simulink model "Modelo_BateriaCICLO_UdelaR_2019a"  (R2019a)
settings: Solver=VariableStepAuto  StartTime=0.0  StopTime=inf  RelTol=1e-3
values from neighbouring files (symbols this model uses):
  a = x(1)    [Cycling_LiFePO4.m]    (also in Parametros_A123.m = 2.09162011618e-08; Parametros_A123_pack.m = 2.09162011618e-08)
  A = @(x) x(1)    [Cycling_LiFePO4.m]    (also in LMFsolve.m = J'*J; Parametros_A123.m = 0.3446; Parametros_A123_pack.m = 0.3446)
  Alpha = 1093.6    [Parametros_A123.m]    (also in Parametros_A123_pack.m)
  b = x(2)    [Cycling_LiFePO4.m]    (also in Parametros_A123.m = -1.21794950859e-05; Parametros_A123_pack.m = -1.21794950859e-05)
  B = @(x) x(2)    [Cycling_LiFePO4.m]    (also in Parametros_A123.m = 13.0435; Parametros_A123_pack.m = 13.0435)
  Beta = 8390.6    [Parametros_A123.m]    (also in Parametros_A123_pack.m)
  c = x(3)    [Cycling_LiFePO4.m]    (also in Parametros_A123.m = 0.00180276688394; Parametros_A123_pack.m = 0.00180276688394)
  Cpol = 0    [Parametros_A123.m]    (also in Parametros_A123_pack.m)
  d = x(4)    [Cycling_LiFePO4.m]    (also in LMFsolve.m = (A+l*D)\v; Parametros_A123.m = -1.70817769928e-06; Parametros_A123_pack.m = -1.70817769928e-06)
  dE_dT = 0.000010001    (= 1.0001e-05)    [Parametros_A123.m]    (also in Parametros_A123_pack.m)
  dQ_dT = 0.0037    [Parametros_A123.m]    (also in Parametros_A123_pack.m)
  Eo = 3.3678    [Parametros_A123.m]    (also in Parametros_A123_pack.m)
  f = x(1)*Q0    [Calendar_LiFePO4.m]    (also in Cycling_LiFePO4.m = f*(exp(g)-1)/(g*exp(0.5)); LMFsolve.m = '; Parametros_A123.m = 5980801.16971; Parametros_A123_pack.m = 5980801.16971)
  g = x(2)    [Calendar_LiFePO4.m]    (also in Cycling_LiFePO4.m = 0.689770643187; Parametros_A123.m = 0.689770643187; Parametros_A123_pack.m = 0.689770643187)
  h = x(3)    [Calendar_LiFePO4.m]    (also in Cycling_LiFePO4.m = -6464.71191685; Parametros_A123.m = -6464.71191685; Parametros_A123_pack.m = -6464.71191685)
  K = 0.0029    [Parametros_A123.m]    (also in Parametros_A123_pack.m)
  Kc = 0.1    [Parametros_A123.m]    (also in Parametros_A123_pack.m)
  Np = 1    [Parametros_A123.m]    (also in Parametros_A123_pack.m = 10)
  Ns = 1    [Parametros_A123.m]    (also in Parametros_A123_pack.m = 200)
  Q = zeros(9,12)    [Calendar_LiFePO4.m]    (also in Cycling_LiFePO4.m = transpose(Q); Parametros_A123.m = 2.3; Parametros_A123_pack.m = 2.3)
  Rohm = 0.01    [Parametros_A123.m]    (also in Parametros_A123_pack.m)
  Rout = 0.6    [Parametros_A123.m]    (also in Parametros_A123_pack.m)
  SOC0 = 100    [Parametros_A123.m]    (also in Parametros_A123_pack.m)
  Ta = 45    [Parametros_A123.m]    (also in Parametros_A123_pack.m = 25)
  Tcrit = 65    [Parametros_A123.m]    (also in Parametros_A123_pack.m)
  Tf = 10    [Parametros_A123.m]    (also in Parametros_A123_pack.m)
  To = 298.15    [Parametros_A123.m]    (also in Parametros_A123_pack.m)
  Tth = 1000    [Parametros_A123.m]    (also in Parametros_A123_pack.m)
  w = 1.5    [Parametros_A123.m]    (also in Parametros_A123_pack.m)
undefined symbols (not defined in the file or in its folder): blocks, Continuous, kV, MW, nthroot, powergui, ZData
libraries: powerlib x8, simulink x3, simulink_extras x1

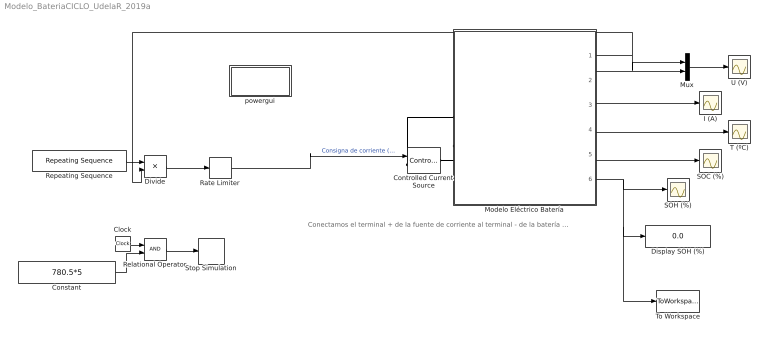
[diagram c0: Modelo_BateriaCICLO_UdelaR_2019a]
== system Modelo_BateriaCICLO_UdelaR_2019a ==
  note: Conectamos el terminal + de la fuente de corriente al terminal - de la batería y viceversa porque consideramos i > 0 durante la descarga.
  Clock : Clock
  Constant : Constant  Value=780.5*5
  Controlled Current Source : powerlib/Electrical Sources/Controlled Current Source  Initialize=on  Source_Type=AC  Amplitude=0  Phase=0  Frequency=0  Measurements=None
  Display SOH (%) : Display
  Divide : Product  Inputs=*/
  I (A) : Scope
  Modelo Eléctrico Batería : Subsystem  VariantControl=Continuous
  Mux : Mux  Inputs=2
  Rate Limiter : RateLimiter  RisingSlewLimit=inf  FallingSlewLimit=-inf  SampleTimeMode=inherited
  Relational Operator : RelationalOperator  OutDataTypeStr=boolean  RndMeth=Simplest
  Repeating Sequence : simulink/Sources/Repeating Sequence  rep_seq_t=t  rep_seq_y=P
  SOC (%) : Scope
  SOH (%) : Scope
  Stop Simulation : Stop
  T (ºC) : Scope
  To Workspace : ToWorkspace  VariableName=SOH  SampleTime=7000
  U (V) : Scope
  powergui : Subsystem  Priority=1  AncestorBlock=powerlib/powergui  DialogController=POWERSYS.PowerSysDialog  InitFcn=powergui( 'InitFcn_Callback' , gcb , 0 , [ ] );  mask(PSB option menu block){SimulationMode=Continuous, SampleTime=50e-6, frequency=60, Iterations=50, frequencyindice=0, Pbase=100e6, ErrMax=1e-4, UnitsV=kV, UnitsW=MW, buscounter=0, FunctionMessages=off, echomessages=off, EnableUseOfTLC=off, CurrentSourceSwitches=off, DisableSnubberDevices=off, DisableRonSwitches=off, DisableVfSwitches=off, DisplayEquations=off, AutomaticDiscreteSolvers=off, SolverType=Tustin/Backward Euler (TBE), Interpol=off, ExternalGateDelay=off, methode=off, Ts=100, x0status=blocks, SPID=on, SwTol=0, HookPort=off, NonlinearTolerance=1e-4, nMaxIteration=100, ContinueOnMaxIteration=off, RestoreLinks=warning, ResistiveCurrentMeasurement=off, Frange=[0:2:500], Ylog=off, Xlog=on, ShowGrid=off, save=off, variable=ZData, structure=0, ZoomFFT=off, StartTime=0.0, cycles=1, DisplayStyle=1, fundamental=60, FreqAxis=off, MaxFrequency=1000, frequencyindicesteady=1, RmsSteady=1, display=off}
      mask prompts: SimulationMode "Simulation type:"; SampleTime "Sample time (s):"; frequency "Frequency (Hz):"; Iterations "Max iterations"; frequencyindice "Frequency (Hz)"; Pbase "Base power (VA)"; ErrMax "PQ tolerance (pu)"; UnitsV "Voltage units"; UnitsW "Power units"; buscounter "Load flow bus counter"; FunctionMessages "Disable Specialized Power Systems warnings"; echomessages "Display Specialized Power Systems compilation messages"; EnableUseOfTLC "Use TLC file when in Accelerator Simulation Mode and for code generation"; CurrentSourceSwitches "Disable ideal switching"; DisableSnubberDevices "Disable snubbers in switching devices"; DisableRonSwitches "Disable Ron resistances in switching devices"; DisableVfSwitches "Disable forward voltages in switching devices"; DisplayEquations "Display circuit differential equations"; AutomaticDiscreteSolvers "Automatically handle Discrete solver and Advanced tab solver settings of blocks"; SolverType "Discrete solver"; Interpol "Interpolate switching events"; ExternalGateDelay "Use time-stamped gate signals"; methode "Store switching topologies"; Ts "Buffer size (MBytes):"; x0status "Start simulation with initial electrical states from:"; SPID "Use ideal switching devices"; SwTol "Switch tolerance"; HookPort "Allow multiple powergui blocks"; NonlinearTolerance "Solver tolerance"; nMaxIteration "Maximum number of iterations"; ContinueOnMaxIteration "Continue Simulation if maximum number of iterations is reached"; RestoreLinks "Restore disabled links of Simscape Power Systems ST blocks:"; ResistiveCurrentMeasurement "Use non ideal current measurement blocks (1e-4Ohm internal resistance)"; Frange "Frequency Range"; Ylog "Log impedance"; Xlog "log Frequency"; ShowGrid "grid"; save "Save Data To Workspace"; variable "Variable Name"; structure "Structure Name (PSBFFTSCOPE)"; ZoomFFT "ZoomFFT (PSBFFTSCOPE)"; StartTime "Start Time (PSBFFTSCOPE)"; cycles "Cycles (PSBFFTSCOPE)"; DisplayStyle "Display style (PSBFFTSCOPE)"; fundamental "Fundamental (PSBFFTSCOPE)"; FreqAxis "Frequency Axis (PSBFFTSCOPE)"; MaxFrequency "Max Frequency (PSBFFTSCOPE)"; frequencyindicesteady "Frequency indice (STEADYSTATE)"; RmsSteady "RMS display (STEADYSTATE)"; display "Display Results"
      mask help: Set simulation type, simulation parameters, and preferences.
      mask init:
      | dispMessage = powergui('MaskInitialization',gcb,SimulationMode,SampleTime);
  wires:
  Rate Limiter/1 -> Controlled Current Source/1  "Consigna de corriente (A)"
  Modelo Eléctrico Batería/5(SOC) -> SOC (%)/1
  Modelo Eléctrico Batería/6(SOH) -> SOH (%)/1, To Workspace/1, Display SOH (%)/1
  Modelo Eléctrico Batería/2(E) -> Mux/2
  Modelo Eléctrico Batería/3(I medida) -> I (A)/1
  Modelo Eléctrico Batería/4(T) -> T (ºC)/1
  Modelo Eléctrico Batería/1(U) -> Divide/2, Mux/1
  Mux/1 -> U (V)/1
  Repeating Sequence/1 -> Divide/1
  Divide/1 -> Rate Limiter/1
  Clock/1 -> Relational Operator/1
  Constant/1 -> Relational Operator/2
  Relational Operator/1 -> Stop Simulation/1
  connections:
  Modelo Eléctrico Batería/LConn2 -- Controlled Current Source/RConn1
  Modelo Eléctrico Batería/LConn1 -- Controlled Current Source/LConn1

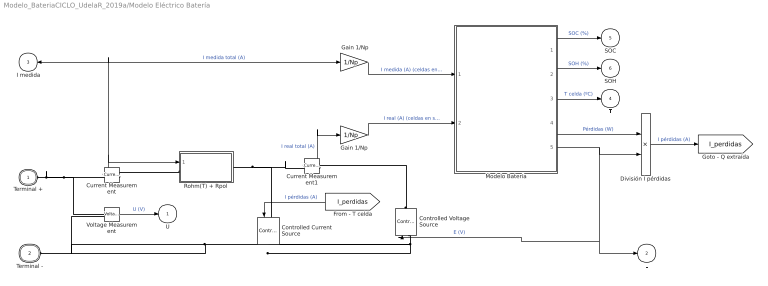
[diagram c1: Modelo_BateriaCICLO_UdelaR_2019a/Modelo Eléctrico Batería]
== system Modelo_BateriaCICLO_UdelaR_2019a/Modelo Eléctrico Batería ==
  "  Gain 1/Np " : Gain  Gain=1/Np
  " Gain 1/Np " : Gain  Gain=1/Np
  Controlled Current Source : powerlib/Electrical Sources/Controlled Current Source  Initialize=on  Source_Type=AC  Amplitude=0  Phase=0  Frequency=0  Measurements=None
  Controlled Voltage Source : powerlib/Electrical Sources/Controlled Voltage Source  Initialize=on  Source_Type=AC  Amplitude=0  Phase=0  Frequency=0  Measurements=None
  Current Measurement : powerlib/Measurements/Current Measurement  PhasorSimulation=off  OutputType=Complex  PSBequivalent=0
  Current Measurement1 : powerlib/Measurements/Current Measurement  PhasorSimulation=off  OutputType=Complex  PSBequivalent=0
  División I pérdidas : Product  Inputs=*/
  Modelo Batería : Subsystem  VariantControl=Continuous
  Rohm(T) + Rpol : Subsystem  VariantControl=Continuous
  Voltage Measurement : powerlib/Measurements/Voltage Measurement  PhasorSimulation=off  OutputType=Complex  PSBequivalent=0
  Terminal + : PMIOPort  Side=Left
  Terminal - : PMIOPort  Port=2  Side=Left
  U : Outport  VectorParamsAs1DForOutWhenUnconnected=off
  E : Outport  Port=2  VectorParamsAs1DForOutWhenUnconnected=off
  I medida : Outport  Port=3  VectorParamsAs1DForOutWhenUnconnected=off
  T : Outport  Port=4  VectorParamsAs1DForOutWhenUnconnected=off
  SOC : Outport  Port=5  VectorParamsAs1DForOutWhenUnconnected=off
  SOH : Outport  Port=6  VectorParamsAs1DForOutWhenUnconnected=off
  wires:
  Voltage Measurement/1 -> U/1  "U (V)"
  Current Measurement/1 -> "  Gain 1/Np "/1, I medida/1, Rohm(T) + Rpol/1(I medida)  "I medida total (A)"
  Current Measurement1/1 -> " Gain 1/Np "/1  "I real total (A)"
  [I_perdidas] -> Controlled Current Source/1  "I pérdidas (A)"
  Modelo Batería/1(SOC) -> SOC/1  "SOC (%)"
  Modelo Batería/2(SOH) -> SOH/1  "SOH (%)"
  Modelo Batería/3(T) -> T/1  "T celda (ºC)"
  Modelo Batería/5(E) -> División I pérdidas/2, Controlled Voltage Source/1, E/1  "E (V)"
  Modelo Batería/4(P Temp) -> División I pérdidas/1  "Pérdidas (W)"
  División I pérdidas/1 -> [I_perdidas]  "I pérdidas (A)"
  " Gain 1/Np "/1 -> Modelo Batería/2(I real)  "I real (A) (celdas en serie)"
  "  Gain 1/Np "/1 -> Modelo Batería/1(I medida)  "I medida (A) (celdas en serie)"
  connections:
  Terminal +/RConn1 -- Voltage Measurement/LConn1 -- Current Measurement/RConn1
  Controlled Voltage Source/LConn1 -- Controlled Current Source/RConn1 -- Voltage Measurement/LConn2 -- Terminal -/RConn1
  Current Measurement/LConn1 -- Rohm(T) + Rpol/LConn1
  Rohm(T) + Rpol/RConn1 -- Controlled Current Source/LConn1 -- Current Measurement1/RConn1
  Controlled Voltage Source/RConn1 -- Current Measurement1/LConn1

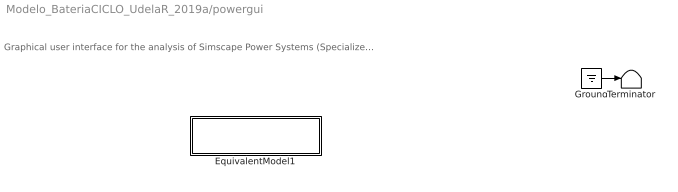
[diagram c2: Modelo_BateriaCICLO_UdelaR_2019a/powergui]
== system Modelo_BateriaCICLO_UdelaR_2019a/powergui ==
  note: Graphical user interface for the analysis of Simscape Power Systems (Specialized Technology) circuits. Place the Powergui block in the top-level of your model and double-click on it to open the GUI.
  EquivalentModel1 : Subsystem
      mask init:
      | S  = GetDataForEquivalentModel('SPID',gcbh,0);
  Ground : Ground
  Terminator : Terminator
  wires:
  Ground/1 -> Terminator/1

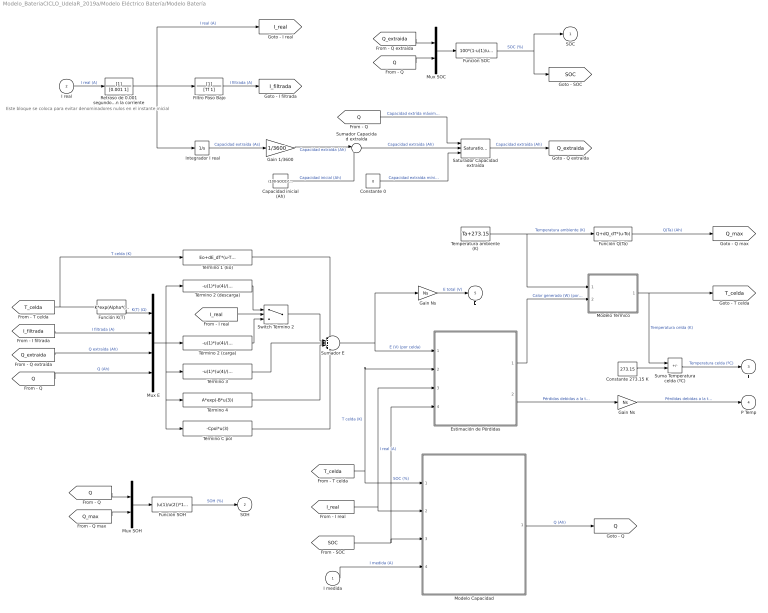
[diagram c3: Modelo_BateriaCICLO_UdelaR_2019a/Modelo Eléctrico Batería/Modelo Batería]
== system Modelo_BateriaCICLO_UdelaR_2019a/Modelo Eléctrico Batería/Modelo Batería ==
  note: Este bloque se coloca para evitar denominadores nulos en el instante inicial
  I medida : Inport
  I real : Inport  Port=2
  " Gain Ns  " : Gain  Gain=Ns
  " Integrador I real" : Integrator
  Capacidad inicial (Ah) : Constant  Value=(100-SOC0)*Q/100
  Constante 0 : Constant  Value=0
  Constante 273.15 K : Constant  Value=273.15
  Estimación de Pérdidas : Subsystem
  Filtro Paso Bajo : TransferFcn  Denominator=[Tf 1]
  Función K(T) : Fcn  Expr=K*exp(Alpha*((1/u)-(1/To)))
  Función Q(Ta) : Fcn  Expr=Q+dQ_dT*(u-To)
  Función SOC : Fcn  Expr=100*(1-u(1)/u(2))
  Función SOH : Fcn  Expr=(u(1)/u(2))*100
  Gain 1/3600 : Gain  Gain=1/3600
  Gain Ns : Gain  Gain=Ns
  Modelo Capacidad : Subsystem  VariantControl=Continuous
  Modelo Térmico : Subsystem  VariantControl=Continuous
  Mux E : Mux
  Mux SOC : Mux  Inputs=2
  Mux SOH : Mux  Inputs=2
  Retraso de 0.001 segundos en la corriente : TransferFcn  Denominator=[0.001 1]
  Saturador Capacidad extraída : simulink/Discontinuities/Saturation Dynamic  OutMin=[]  OutMax=[]  OutDataTypeStr=Inherit: Same as second input  OutDataType=fixdt(1, 16)  OutScaling=2^-10  DoSatur=off
  Suma Temperatura celda (ºC) : Sum  Inputs=+-
  Sumador Capacidad extraída : Sum  Inputs=|++
  Sumador E : Sum  Inputs=+++++
  Switch Término 2 : Switch  Criteria=u2 > Threshold
  Temperatura ambiente (K) : Constant  Value=Ta+273.15
  Término 1 (Eo) : Fcn  Expr=Eo+dE_dT*(u-To)
  Término 2 (carga) : Fcn  Expr=-u(1)*(u(4)/(u(3)+Kc*u(4)))*u(2)
  Término 2 (descarga) : Fcn  Expr=-u(1)*(u(4)/(u(4)-u(3)))*u(2)
  Término 3 : Fcn  Expr=-u(1)*(u(4)/(u(4)-u(3)))*u(3)
  Término 4 : Fcn  Expr=A*exp(-B*u(3))
  Término C pol : Fcn  Expr=-Cpol*u(3)
  SOC : Outport  VectorParamsAs1DForOutWhenUnconnected=off
  SOH : Outport  Port=2  VectorParamsAs1DForOutWhenUnconnected=off
  T : Outport  Port=3  VectorParamsAs1DForOutWhenUnconnected=off
  P Temp : Outport  Port=4  VectorParamsAs1DForOutWhenUnconnected=off
  E : Outport  Port=5  VectorParamsAs1DForOutWhenUnconnected=off
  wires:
  Filtro Paso Bajo/1 -> [I_filtrada]  "I filtrada (A)"
  " Integrador I real"/1 -> Gain 1/3600/1  "Capacidad extraída (As)"
  [Q] -> Saturador Capacidad extraída/1  "Capacidad extrída máxima (Ah)"
  Constante 0/1 -> Saturador Capacidad extraída/3  "Capacidad extraída mínima (Ah)"
  Saturador Capacidad extraída/1 -> [Q_extraida]  "Capacidad extraída (Ah)"
  [T_celda] -> Término 1 (Eo)/1, Función K(T)/1  "T celda (K)"
  Función K(T)/1 -> Mux E/1  "K(T) (Ω)"
  [I_filtrada] -> Mux E/2  "I filtrada (A)"
  [Q_extraida] -> Mux E/3  "Q extraída (Ah)"
  [Q] -> Mux E/4  "Q (Ah)"
  Término 2 (descarga)/1 -> Switch Término 2/1
  Término 2 (carga)/1 -> Switch Término 2/3
  [I_real] -> Switch Término 2/2
  Término 4/1 -> Sumador E/4
  Switch Término 2/1 -> Sumador E/2
  Mux E/1 -> Término 4/1, Término C pol/1, Término 3/1, Término 2 (descarga)/1, Término 2 (carga)/1
  Término 1 (Eo)/1 -> Sumador E/1
  Sumador E/1 -> Gain Ns/1, Estimación de Pérdidas/1(E)  "E (V) (por celda)"
  Estimación de Pérdidas/2(P Temp) -> " Gain Ns  "/1  "Pérdidas debidas a la temperatura (W) (por celda)"
  " Gain Ns  "/1 -> P Temp/1  "Pérdidas debidas a la temperatura (W) (celdas en serie)"
  Estimación de Pérdidas/1(H) -> Modelo Térmico/2(H)  "Calor generado (W) (por celda)"
  Temperatura ambiente (K)/1 -> Función Q(Ta)/1, Modelo Térmico/1(Ta)  "Temperatura ambiente (K)"
  Función Q(Ta)/1 -> [Q_max]  "Q(Ta) (Ah)"
  Modelo Térmico/1(T) -> [T_celda], Suma Temperatura celda (ºC)/1  "Temperatura celda (K)"
  Suma Temperatura celda (ºC)/1 -> T/1  "Temperatura celda (ºC)"
  Constante 273.15 K/1 -> Suma Temperatura celda (ºC)/2
  [Q_extraida] -> Mux SOC/1
  [Q] -> Mux SOC/2
  [Q] -> Mux SOH/1
  [Q_max] -> Mux SOH/2
  Mux SOH/1 -> Función SOH/1
  Mux SOC/1 -> Función SOC/1
  Función SOH/1 -> SOH/1  "SOH (%)"
  Función SOC/1 -> SOC/1, [SOC]  "SOC (%)"
  Modelo Capacidad/1(Q) -> [Q]  "Q (Ah)"
  Gain Ns/1 -> E/1  "E total (V)"
  Retraso de 0.001 segundos en la corriente/1 -> " Integrador I real"/1, [I_real], Filtro Paso Bajo/1  "I real (A)"
  Gain 1/3600/1 -> Sumador Capacidad extraída/1  "Capacidad extraída (Ah)"
  Capacidad inicial (Ah)/1 -> Sumador Capacidad extraída/2  "Capacidad inicial (Ah)"
  Sumador Capacidad extraída/1 -> Saturador Capacidad extraída/2  "Capacidad extraída (Ah)"
  Término 3/1 -> Sumador E/3
  Término C pol/1 -> Sumador E/5
  [T_celda] -> Estimación de Pérdidas/2(T), Modelo Capacidad/1(T)  "T celda (K)"
  [I_real] -> Estimación de Pérdidas/3(I real), Modelo Capacidad/2(I real)  "I real (A)"
  [SOC] -> Estimación de Pérdidas/4(SOC), Modelo Capacidad/3(SOC)  "SOC (%)"
  I real/1 -> Retraso de 0.001 segundos en la corriente/1  "I real (A)"
  I medida/1 -> Modelo Capacidad/4(I medida)  "I medida (A)"

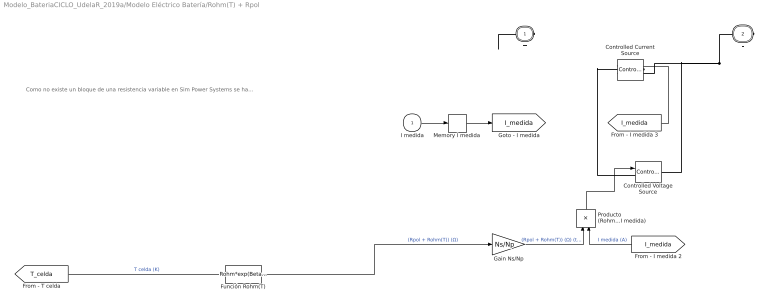
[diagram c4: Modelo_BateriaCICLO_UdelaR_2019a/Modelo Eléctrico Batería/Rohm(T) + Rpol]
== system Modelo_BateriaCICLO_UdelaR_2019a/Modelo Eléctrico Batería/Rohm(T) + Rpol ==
  note: Como no existe un bloque de una resistencia variable en Sim Power Systems se ha recreado una. Para ello se se coloca en bornes del bloque una tensión igual a la resistencia deseada y se multiplica por la corriente que circula por ella. Por lo tanto, el cociente de U/I obtenido es igual a R. Nótese que la polarización de los términales es la inversa, esto se debe a que se ha considerado que la corriente durante la descarga es i > 0.
  I medida : Inport
  Controlled Current Source : powerlib/Electrical Sources/Controlled Current Source  Initialize=on  Source_Type=AC  Amplitude=0  Phase=0  Frequency=0  Measurements=None
  Controlled Voltage Source : powerlib/Electrical Sources/Controlled Voltage Source  Initialize=on  Source_Type=AC  Amplitude=0  Phase=0  Frequency=0  Measurements=None
  Función Rohm(T) : Fcn  Expr=Rohm*exp(Beta*((1/u)-(1/To)))
  Gain Ns/Np : Gain  Gain=Ns/Np
  Memory I medida : Memory
  "Producto (Rohm+Rpol)*(I medida) " : Product
  + : PMIOPort  Side=Left
  - : PMIOPort  Port=2  Side=Right
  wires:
  [T_celda] -> Función Rohm(T)/1  "T celda (K)"
  "Producto (Rohm+Rpol)*(I medida) "/1 -> Controlled Voltage Source/1
  Función Rohm(T)/1 -> Gain Ns/Np/1  "(Rpol + Rohm(T)) (Ω)"
  [I_medida] -> "Producto (Rohm+Rpol)*(I medida) "/2  "I medida (A)"
  [I_medida] -> Controlled Current Source/1
  Gain Ns/Np/1 -> "Producto (Rohm+Rpol)*(I medida) "/1  "(Rpol + Rohm(T)) (Ω) (total de la batería)"
  I medida/1 -> Memory I medida/1
  Memory I medida/1 -> [I_medida]
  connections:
  -/RConn1 -- Controlled Voltage Source/RConn1 -- Controlled Current Source/LConn1
  Controlled Current Source/RConn1 -- Controlled Voltage Source/LConn1 -- +/RConn1

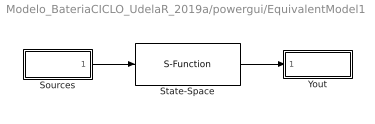
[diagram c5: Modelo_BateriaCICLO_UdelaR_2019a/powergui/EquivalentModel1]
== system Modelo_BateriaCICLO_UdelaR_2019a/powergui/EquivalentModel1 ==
  Sources : Subsystem
  State-Space : S-Function  FunctionName=sfun_spid_contc  Parameters=S.Mg, [S.nb.x S.nb.u S.nb.y S.nb.s], S.x0, S.MgColNames  SFunctionDeploymentMode=off  EnableBusSupport=off
  Yout : Subsystem
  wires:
  State-Space/1 -> Yout/1(v,i)
  Sources/1(u) -> State-Space/1

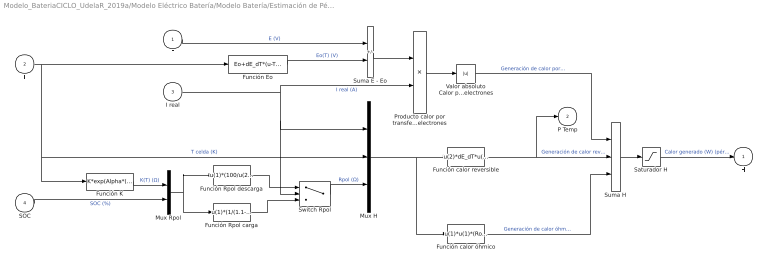
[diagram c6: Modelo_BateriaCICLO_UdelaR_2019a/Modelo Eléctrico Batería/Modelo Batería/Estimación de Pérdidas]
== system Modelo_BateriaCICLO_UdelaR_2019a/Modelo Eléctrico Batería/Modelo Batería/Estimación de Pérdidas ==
  E : Inport
  T : Inport  Port=2
  I real : Inport  Port=3
  SOC : Inport  Port=4
  Función Eo : Fcn  Expr=Eo+dE_dT*(u-To)
  Función K : Fcn  Expr=K*exp(Alpha*((1/u)-(1/To)))
  Función Rpol carga : Fcn  Expr=u(1)*(1/(1.1-(u(2)/100)))
  Función Rpol descarga : Fcn  Expr=u(1)*(100/u(2))
  Función calor reversible : Fcn  Expr=u(2)*dE_dT*u(1)
  Función calor óhmico : Fcn  Expr=u(1)*u(1)*(Rohm*exp(Beta*((1/u(2))-(1/To)))+u(3))
  Mux H : Mux  Inputs=3
  Mux Rpol : Mux  Inputs=2
  Producto calor por transferencia de electrones : Product
  Saturador H : Saturate  UpperLimit=inf  LowerLimit=0
  Suma E - Eo : Sum  Inputs=-+
  Suma H : Sum  Inputs=+++
  Switch Rpol : Switch  Criteria=u2 > Threshold
  Valor absoluto Calor por transferencia de electrones : Abs
  H : Outport  VectorParamsAs1DForOutWhenUnconnected=off
  P Temp : Outport  Port=2  VectorParamsAs1DForOutWhenUnconnected=off
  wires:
  Función calor óhmico/1 -> Suma H/3  "Generación de calor óhmica (W) (pérdidas)"
  Función calor reversible/1 -> Suma H/2, P Temp/1  "Generación de calor reversible (W) (pérdidas)"
  Valor absoluto Calor por transferencia de electrones/1 -> Suma H/1  "Generación de calor por transferencia de electrones (W) (pérdidas)"
  Saturador H/1 -> H/1  "Calor generado (W) (pérdidas)"
  Función Rpol descarga/1 -> Switch Rpol/1
  Mux H/1 -> Función calor óhmico/1, Función calor reversible/1
  I real/1 -> Producto calor por transferencia de electrones/2, Switch Rpol/2, Mux H/1  "I real (A)"
  T/1 -> Función Eo/1, Función K/1, Mux H/2  "T celda (K)"
  Función Eo/1 -> Suma E - Eo/2  "Eo(T) (V)"
  E/1 -> Suma E - Eo/1  "E (V)"
  Suma E - Eo/1 -> Producto calor por transferencia de electrones/1
  Producto calor por transferencia de electrones/1 -> Valor absoluto Calor por transferencia de electrones/1
  Switch Rpol/1 -> Mux H/3  "Rpol (Ω)"
  Mux Rpol/1 -> Función Rpol carga/1, Función Rpol descarga/1
  Función K/1 -> Mux Rpol/1  "K(T) (Ω)"
  SOC/1 -> Mux Rpol/2  "SOC (%)"
  Suma H/1 -> Saturador H/1
  Función Rpol carga/1 -> Switch Rpol/3

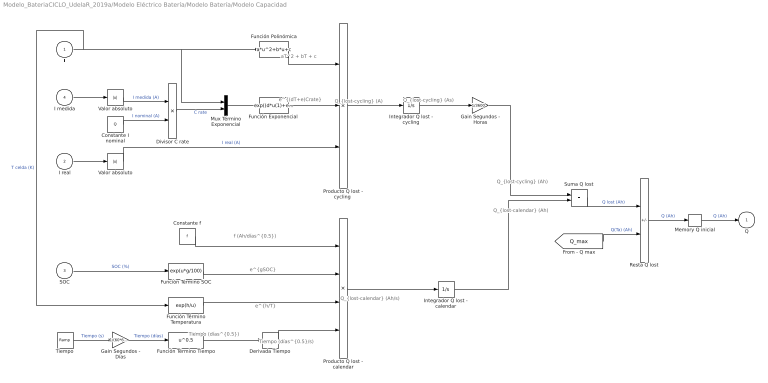
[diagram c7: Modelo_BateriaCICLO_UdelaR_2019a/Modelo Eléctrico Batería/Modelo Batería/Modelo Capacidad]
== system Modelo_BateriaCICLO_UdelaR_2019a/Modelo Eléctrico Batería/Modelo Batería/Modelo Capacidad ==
  note: aT^2 + bT + c
  note: e^{(dT+e)Crate}
  note: Q_{lost-cycling} (A)
  note: Q_{lost-cycling} (As)
  note: Q_{lost-cycling} (Ah)
  note: Tiempo (días^{0.5})
  note: e^{gSOC}
  note: e^{h/T}
  note: f (Ah/días^{0.5})
  note: Tiempo (días^{0.5}/s)
  note: Q_{lost-calendar} (Ah/s)
  note: Q_{lost-calendar} (Ah)
  T : Inport
  I real : Inport  Port=2
  SOC : Inport  Port=3
  I medida : Inport  Port=4
  " Valor absoluto " : Abs
  Constante I nominal : Constant  Value=Q
  Constante f : Constant  Value=f
  Derivada Tiempo : Derivative
  Divisor C rate : Product  Inputs=*/
  "Función Exponencial " : Fcn  Expr=exp((d*u(1)+e)*u(2))
  Función Polinómica : Fcn  Expr=a*u^2+b*u+c
  Función Término SOC : Fcn  Expr=exp(u*g/100)
  Función Término Temperatura : Fcn  Expr=exp(h/u)
  Función Término Tiempo : Fcn  Expr=u^0.5
  Gain Segundos - Días : Gain  Gain=1/(60*60*24)
  Gain Segundos - Horas : Gain  Gain=1/3600
  Integrador Q lost - calendar : Integrator
  Integrador Q lost - cycling : Integrator
  Memory Q inicial : Memory  InitialCondition=Q
  Mux Término Exponencial : Mux  Inputs=2
  Producto Q lost - calendar : Product  Inputs=4
  "Producto Q lost - cycling " : Product  Inputs=3
  Resta Q lost : Sum  Inputs=-+
  Suma Q lost : Sum
  Tiempo : simulink/Sources/Ramp  slope=12/w  start=0  InitialOutput=0
  Valor absoluto : Abs
  Q : Outport  VectorParamsAs1DForOutWhenUnconnected=off
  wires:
  Memory Q inicial/1 -> Q/1  "Q (Ah)"
  Resta Q lost/1 -> Memory Q inicial/1  "Q (Ah)"
  Constante I nominal/1 -> Divisor C rate/2  "I nominal (A)"
  I real/1 -> " Valor absoluto "/1
  Divisor C rate/1 -> Mux Término Exponencial/2  "C rate"
  [Q_max] -> Resta Q lost/2  "Q(Ta) (Ah)"
  Función Término SOC/1 -> Producto Q lost - calendar/2
  Gain Segundos - Días/1 -> Función Término Tiempo/1  "Tiempo (días)"
  Producto Q lost - calendar/1 -> Integrador Q lost - calendar/1
  SOC/1 -> Función Término SOC/1  "SOC (%)"
  "Producto Q lost - cycling "/1 -> Integrador Q lost - cycling/1
  Integrador Q lost - cycling/1 -> Gain Segundos - Horas/1
  T/1 -> Mux Término Exponencial/1, Función Polinómica/1, Función Término Temperatura/1  "T celda (K)"
  Función Término Tiempo/1 -> Derivada Tiempo/1
  Constante f/1 -> Producto Q lost - calendar/1
  Derivada Tiempo/1 -> Producto Q lost - calendar/4
  " Valor absoluto "/1 -> "Producto Q lost - cycling "/3  "I real (A)"
  I medida/1 -> Valor absoluto/1
  Valor absoluto/1 -> Divisor C rate/1  "I medida (A)"
  Mux Término Exponencial/1 -> "Función Exponencial "/1
  Función Polinómica/1 -> "Producto Q lost - cycling "/1
  "Función Exponencial "/1 -> "Producto Q lost - cycling "/2
  Gain Segundos - Horas/1 -> Suma Q lost/1
  Función Término Temperatura/1 -> Producto Q lost - calendar/3
  Tiempo/1 -> Gain Segundos - Días/1  "Tiempo (s)"
  Integrador Q lost - calendar/1 -> Suma Q lost/2
  Suma Q lost/1 -> Resta Q lost/1  "Q lost (Ah)"

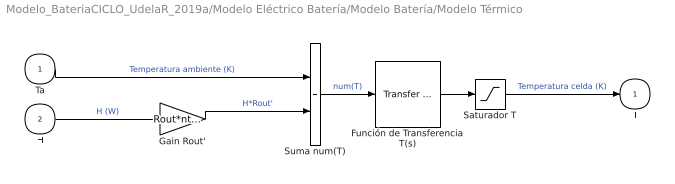
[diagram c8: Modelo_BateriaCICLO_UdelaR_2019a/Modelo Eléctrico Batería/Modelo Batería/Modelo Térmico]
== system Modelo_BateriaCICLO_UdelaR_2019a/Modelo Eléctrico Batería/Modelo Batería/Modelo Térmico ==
  Ta : Inport
  H : Inport  Port=2
  Función de Transferencia T(s) : simulink_extras/Additional Linear/Transfer Fcn (with initial outputs)  N=[1]  D="[Tth  1]"  Y0=Ta+273.15  U0=0
  Gain Rout' : Gain  Gain=Rout*nthroot(0.5*Ns, 6)
  Saturador T : Saturate  UpperLimit=Tcrit+273.15  LowerLimit=0
  Suma num(T) : Sum
  T : Outport  VectorParamsAs1DForOutWhenUnconnected=off
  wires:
  Suma num(T)/1 -> Función de Transferencia T(s)/1  "num(T)"
  Función de Transferencia T(s)/1 -> Saturador T/1
  Gain Rout'/1 -> Suma num(T)/2  "H*Rout'"
  H/1 -> Gain Rout'/1  "H (W)"
  Saturador T/1 -> T/1  "Temperatura celda (K)"
  Ta/1 -> Suma num(T)/1  "Temperatura ambiente (K)"

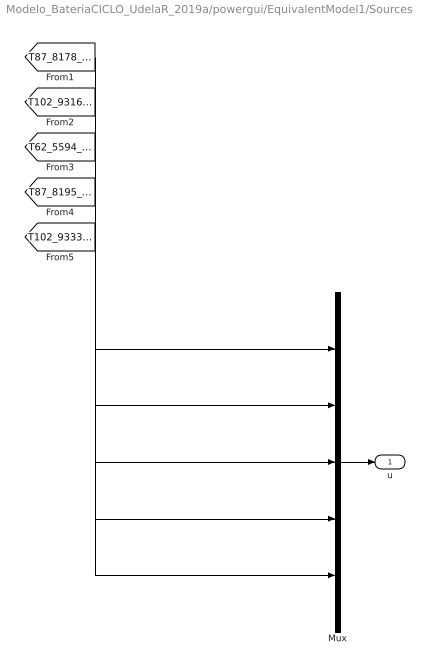
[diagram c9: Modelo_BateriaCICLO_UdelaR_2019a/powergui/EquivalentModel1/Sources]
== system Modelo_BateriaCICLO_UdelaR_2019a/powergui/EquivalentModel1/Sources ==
  Mux : Mux  Inputs=[1 1 1 1 1]
  u : Outport  VectorParamsAs1DForOutWhenUnconnected=off
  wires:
  Mux/1 -> u/1
  [T87_8178_15402510619818] -> Mux/1
  [T102_9316_19639504091308] -> Mux/2
  [T62_5594_6962520765397] -> Mux/3
  [T87_8195_15727979385544] -> Mux/4
  [T102_9333_20055620979228] -> Mux/5

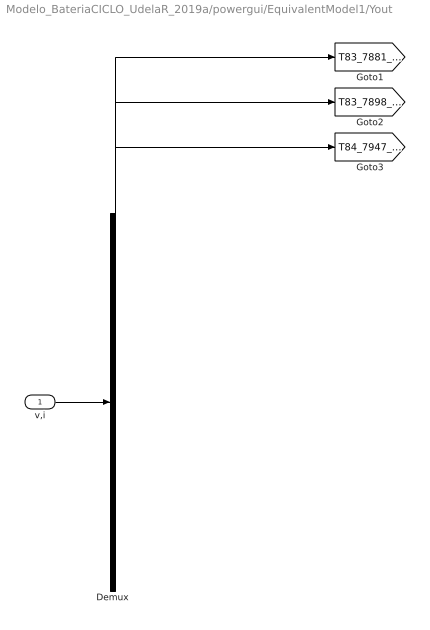
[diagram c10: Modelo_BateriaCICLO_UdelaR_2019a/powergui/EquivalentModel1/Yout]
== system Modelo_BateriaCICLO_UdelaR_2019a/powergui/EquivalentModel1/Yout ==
  v,i : Inport
  Demux : Demux  Outputs=[1 1 1]
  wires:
  v,i/1 -> Demux/1
  Demux/1 -> [T83_7881_15125871722280]
  Demux/2 -> [T83_7898_15350115032313]
  Demux/3 -> [T84_7947_15293716745179]
